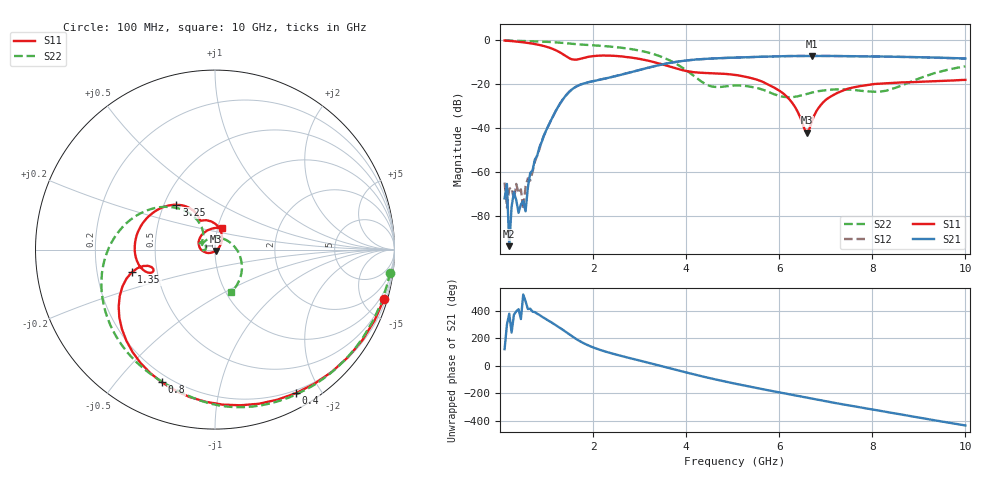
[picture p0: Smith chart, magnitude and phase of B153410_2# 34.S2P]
!  2-Port S-parameters saved by WinCal
! VAR MeasName=S-Parameters (CALIBRATED_DATA) read from VNA (N5245A)
! VAR MeasDate=2016-12-23 10:01:06
! VAR NAME=B153410_2# 34
! VAR FILENAME=B153410_2# 34.S2P
! VAR DATE=2016-12-23 10:01:06
! VAR PHYS_PORTS=1,2
# Hz S DB R 50
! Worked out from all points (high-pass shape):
!   199 points, 100 MHz to 10 GHz, reference 50 ohm
!   highest |S21| = -7.13 dB at 6.7 GHz (marker M1); lowest = -93.5 dB at 200 MHz (marker M2)
!   |S21| within 3 dB of the highest: 3.704 GHz to end of sweep
!   lowest |S11| = -42.1 dB at 6.6 GHz (marker M3), VSWR 1.02, Z = 50.4 - j0.709 ohm
!   |S11| at or under -10 dB: 3.317 GHz to end of sweep
!   |S22| runs from -25.9 to -0.1 dB; largest |S21 - S12| = 0.0031
!   S11 on the Smith chart (normalised r, x): 100 MHz: 0.47, -7.02; 400 MHz: 0.17, -1.70; 800 MHz: 0.16, -0.66; 1.35 GHz: 0.36, -0.12; 3.25 GHz: 0.58, +0.32; 10 GHz: 1.05, +0.25
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1e8  -0.16 -16.2  -71.82 120.6  -64.63 156.2  -0.14 -7.5
1.5e8  -0.24 -23.9  -65.26 -61.6  -76.08 147.2  -0.18 -10.9
2e8  -0.32 -31.5  -93.53 17.0  -67.45 59.7  -0.22 -14.3
3e8  -0.52 -46.3  -69.06 10.0  -72.53 116.9  -0.29 -21.0
3.5e8  -0.63 -53.4  -72.62 34.2  -65.27 -106.3  -0.31 -24.3
4e8  -0.74 -60.5  -78.38 49.5  -69.54 177.3  -0.35 -27.6
4.5e8  -0.86 -67.4  -74.50 -21.9  -67.74 50.4  -0.36 -30.9
5e8  -0.98 -74.2  -73.09 155.5  -76.79 91.8  -0.39 -34.2
5.5e8  -1.12 -80.7  -77.70 107.2  -66.47 34.8  -0.42 -37.5
6.5e8  -1.42 -93.6  -60.32 53.2  -63.79 50.2  -0.49 -44.1
8e8  -1.98 -111.8  -52.46 16.6  -52.30 16.4  -0.59 -53.9
1.35e9  -6.36 -164.8  -27.00 -99.3  -26.93 -99.4  -1.24 -89.2
1.75e9  -8.34 -160.2  -20.03 172.0  -20.02 172.0  -2.01 -111.6
3.25e9  -9.66 130.7  -12.17 17.1  -12.17 17.0  -6.01 160.8
3.4e9  -10.46 125.4  -11.43 4.2  -11.42 4.1  -7.03 151.3
5.05e9  -15.80 100.6  -7.92 -128.9  -7.94 -128.8  -20.59 158.1
6.1e9  -24.45 51.4  -7.26 161.0  -7.27 161.1  -25.74 163.8
6.6e9  -42.07 -63.3  -7.13 128.8  -7.14 128.8  -24.39 -176.4
6.7e9  -36.81 -118.9  -7.13 122.4  -7.14 122.4  -23.85 -176.6
7.25e9  -23.93 -169.4  -7.22 88.2  -7.20 88.2  -22.35 165.2
8.35e9  -19.49 143.1  -7.51 23.1  -7.49 23.0  -22.61 57.1
1e10  -18.03 71.8  -8.35 -71.4  -8.40 -71.3  -11.90 -69.2
